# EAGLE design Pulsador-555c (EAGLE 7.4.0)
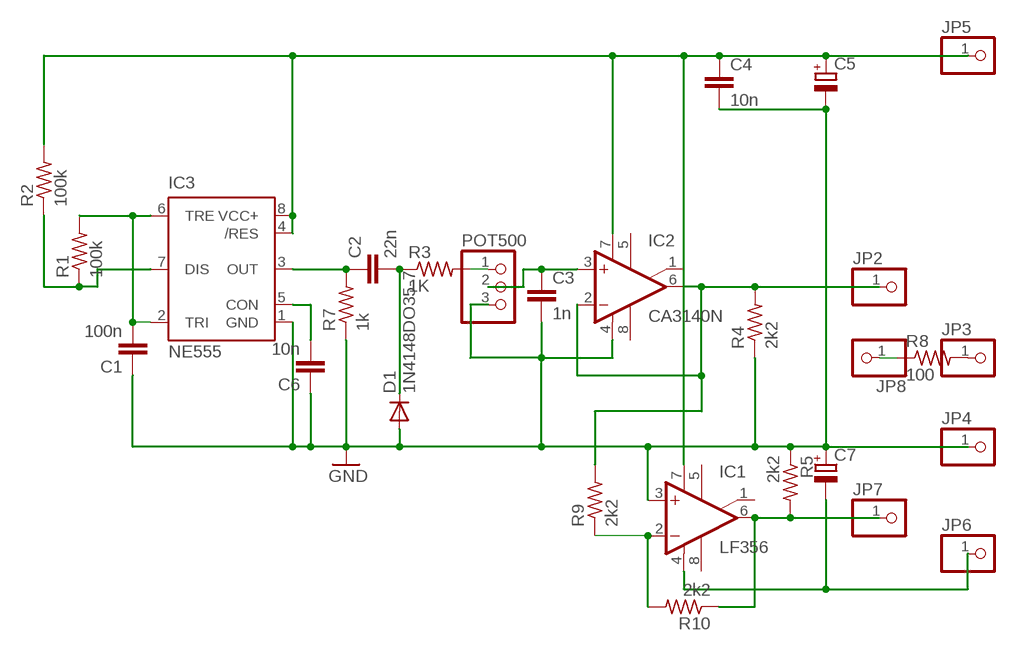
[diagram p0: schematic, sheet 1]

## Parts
C1  100n  C-EU050-024X044  [C050-024X044]
C2  22n  C-EU050-024X044  [C050-024X044]
C3  1n  C-EU050-024X044  [C050-024X044]
C4  10n  C-EU025-025X050  [C025-025X050]
C5  CPOL-EUE2.5-6  [E2,5-6]
C6  10n  C-EU050-024X044  [C050-024X044]
C7  CPOL-EUE2.5-6  [E2,5-6]
D1  1N4148DO35-7  [DO35-7]
IC1  LF356  CA3140N  [DIL08]
IC2  CA3140N  [DIL08]
IC3  NE555  [DIL-08]
JP2  PINHD-1X1  [1X01]
JP3  PINHD-1X1  [1X01]
JP4  PINHD-1X1  [1X01]
JP5  PINHD-1X1  [1X01]
JP6  PINHD-1X1  [1X01]
JP7  PINHD-1X1  [1X01]
JP8  PINHD-1X1  [1X01]
POT500  PINHD-1X3  [1X03]
R1  100k  R-US_0204/7  [0204/7]
R2  100k  R-US_0204/7  [0204/7]
R3  1K  R-US_0204/7  [0204/7]
R4  2k2  R-US_0204/7  [0204/7]
R5  2k2  R-US_0204/7  [0204/7]
R7  1k  R-US_0204/7  [0204/7]
R8  100  R-US_0204/7  [0204/7]
R9  2k2  R-US_0204/7  [0204/7]
R10  2k2  R-US_0204/7  [0204/7]

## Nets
GND: C1.1 C3.2 C4.2 C5.- C6.1 C7.+ D1.A IC1.3(+IN) IC2.4(V-) IC3.1(GND) JP4.1 POT500.3 R4.1 R5.1 R7.1
N$1: IC1.2(-IN) R9.1 R10.2
N$2: C6.2 IC3.5(CON)
N$3: C2.1 IC3.3(OUT) R7.2
N$4: C2.2 D1.C R3.1
N$5: C7.- IC1.4(V-) JP6.1
N$6: POT500.1 R3.2
N$7: IC2.2(-IN) IC2.6(OUT) JP2.1 R4.2 R9.2
N$9: IC3.7(DIS) R1.1 R2.1
N$10: C4.1 C5.+ IC1.7(V+) IC2.7(V+) IC3.4(/RES) IC3.8(VCC+) JP5.1 R2.2
N$11: C1.2 IC3.2(TRI) IC3.6(TRE) R1.2
N$12: JP3.1 R8.2
N$13: IC1.6(OUT) JP7.1 R5.2 R10.1
N$14: JP8.1 R8.1
N$16: C3.1 IC2.3(+IN) POT500.2
Unconnected: IC1.1(ON/CMP) IC1.5(ON) IC1.8(CMP) IC2.1(ON/CMP) IC2.5(ON) IC2.8(CMP)

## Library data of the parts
C1-C4 C6 = rcl:C-EU: CAPACITOR, European symbol
C5 C7 = rcl:CPOL-EU: POLARIZED CAPACITOR, European symbol
D1 = diode:1N4148: DIODE
IC1 IC2 = linear:CA3140: OP AMP
IC3 = st-microelectronics:NE555: General purpose bipolar Timer; MF: Arrow Electronics; MPN: NE555N; OC_FARNELL: 1467742; OC_NEWARK: 89K1486
JP2-JP8 = pinhead:PINHD-1X1: PIN HEADER
POT500 = pinhead:PINHD-1X3: PIN HEADER
R1-R5 R7-R10 = rcl:R-US_: RESISTOR, American symbol

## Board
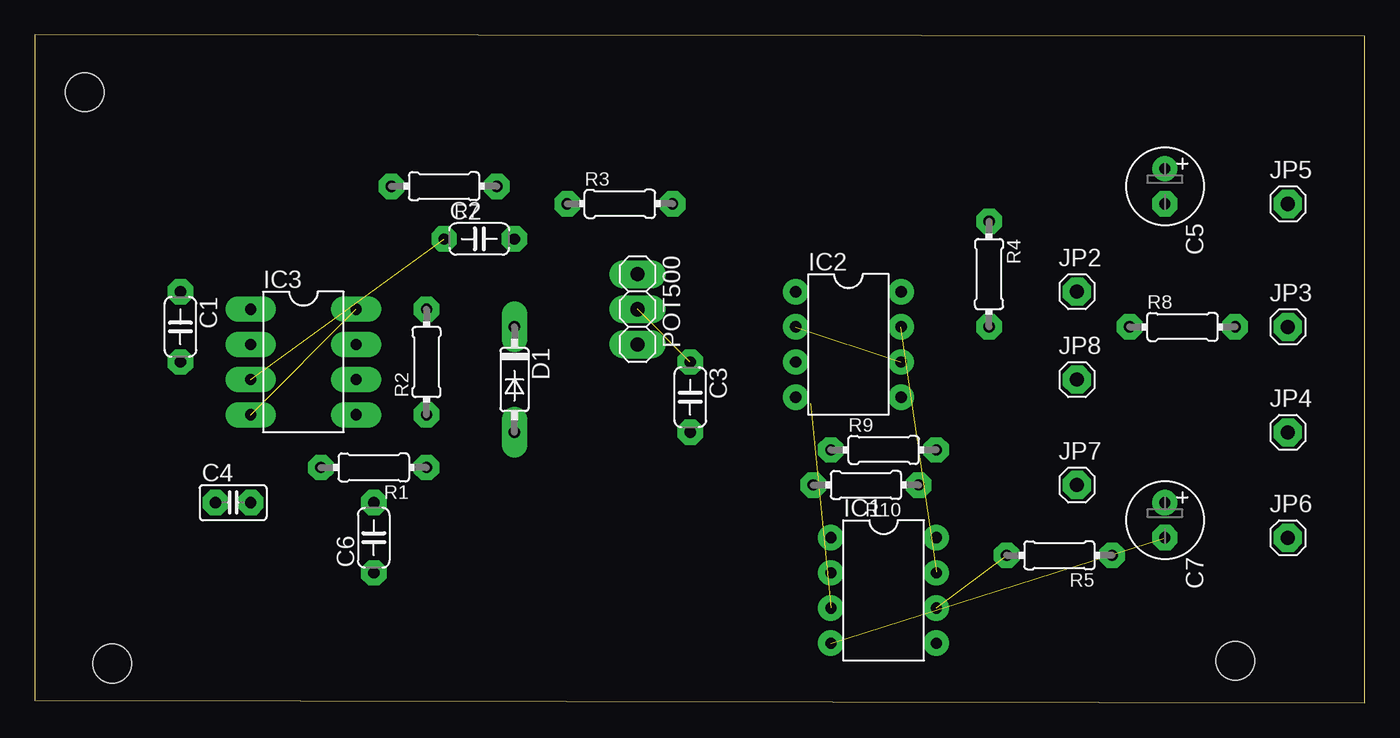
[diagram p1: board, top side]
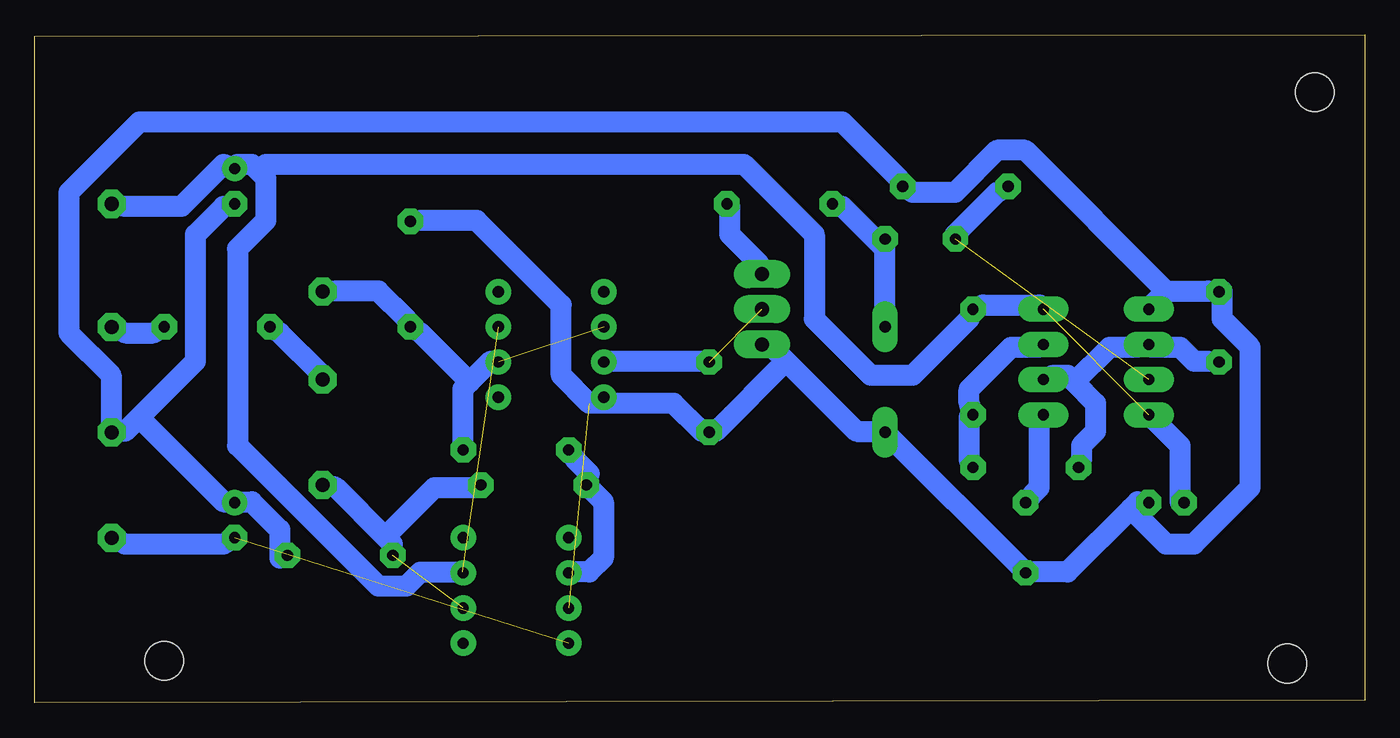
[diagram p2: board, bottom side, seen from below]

Size 96.1 x 48.3 mm. Coordinates in mm from the lower left corner, seen from the top.
Outline: 0,0.2 96.1,0 96.1,48.2 0,48.3 0,0.2
Copper layers (1*16): Top 0.035mm / dielectric 1.5mm / Bottom 0.035mm
Design rules "default *": minimum track width 60mil, minimum drill 24mil, track to track 20mil, track to pad 20mil, pad to pad 8mil, via to via 8mil, smd to smd 8mil, copper to edge 40mil, drill to drill 8mil, minimum pad ring 20mil, minimum via ring 8mil, stop-mask expansion 4mil, vias tented up to drill 0mil, thermal gap 10mil
Holes 2.8 mm at 3.61,44.15 86.73,3.05 5.61,2.85

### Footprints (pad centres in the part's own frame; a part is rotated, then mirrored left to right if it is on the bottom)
C050-024X044 = drill 0.813 octagon: 1 -2.54,0; 2 2.54,0
C025-025X050 = drill 0.813 octagon: 1 -1.27,0; 2 1.27,0
E2,5-6 = drill 0.813 pad 1.6: + -1.27,0 | drill 0.813 pad 1.6 octagon: - 1.27,0
DO35-7 = drill 0.813 long: A 3.81,0; C -3.81,0
DIL08 = drill 0.813 pad 1.27: 1 -3.81,-3.81; 2 -1.27,-3.81; 3 1.27,-3.81; 4 3.81,-3.81; 5 3.81,3.81; 6 1.27,3.81; 7 -1.27,3.81; 8 -3.81,3.81
DIL-08 = drill 0.813 long: 1 -3.81,-3.81; 2 -1.27,-3.81; 3 1.27,-3.81; 4 3.81,-3.81; 5 3.81,3.81; 6 1.27,3.81; 7 -1.27,3.81; 8 -3.81,3.81
1X01 = drill 1.016 octagon: 1 0,0
1X03 = drill 1.016 long: 1 -2.54,0; 2 0,0; 3 2.54,0
0204/7 = drill 0.813 octagon: 1 -3.81,0; 2 3.81,0

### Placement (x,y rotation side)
C1  10.53,27.18 270 top
C2  32.12,33.53 0 top
C3  47.36,22.1 270 top
C4  14.34,14.48 0 top
C5  81.65,37.34 270 top
C6  24.5,11.94 90 top
C7  81.65,13.21 270 top
D1  34.66,23.37 270 top
IC1  61.33,8.13 270 top
IC2  58.79,25.91 270 top
IC3  19.42,24.64 270 top
JP2  75.3,29.72 0 top
JP3  90.54,27.18 0 top
JP4  90.54,19.56 0 top
JP5  90.54,36.07 0 top
JP6  90.54,11.94 0 top
JP7  75.3,15.75 0 top
JP8  75.3,23.37 0 top
POT500  43.55,28.45 270 top
R1  24.5,17.02 180 top
R2  28.31,24.64 90 top
R3  42.28,36.07 0 top
R4  68.95,30.99 270 top
R5  74.03,10.67 180 top
R7  29.58,37.34 180 top
R8  82.92,27.18 0 top
R9  61.33,18.29 0 top
R10  60.06,15.75 180 top

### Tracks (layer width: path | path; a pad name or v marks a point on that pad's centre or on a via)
GND  (1 unrouted)
  Bottom 1.524: R5.1 78.38,10.48 78.38,12.51 80.42,14.54 81.43,14.54 C7.+ 82.45,14.54 88.54,20.64 | 88.54,20.64 89.56,19.62 JP4.1 90.58,19.62 90.58,23.69 93.62,26.74 93.62,36.9 88.54,41.98 37.74,41.98 33.68,37.91 R7.1 32.66,36.9 29.62,36.9 26.57,39.94 24.54,39.94 14.38,29.78 | 88.54,20.64 84.48,24.7 84.48,33.85 82.45,35.88 C5.- | 14.38,29.78 11.33,29.78 C1.1 10.31,29.78 10.31,27.75 8.28,25.72 8.28,15.56 12.34,11.5 14.38,11.5 16.92,14.04 | 14.38,29.78 15.39,28.77 IC3.1 | 24.54,9.46 21.49,9.46 16.92,14.04 | 16.92,14.04 16.41,14.54 C4.2 | 34.7,19.62 36.73,19.62 41.81,24.7 | 41.81,24.7 42.82,25.72 POT500.3 | 41.81,24.7 46.89,19.62 C3.2 47.9,19.62 49.94,21.66 55.02,21.66 | 55.02,21.66 56.03,21.66 58.06,23.69 58.06,28.77 64.16,34.86 68.22,34.86 R4.1 | 55.02,21.66 IC2.4 | 34.7,19.62 24.54,9.46 | 24.54,9.46 C6.1 | 34.7,19.62 D1.A
N$1
  Bottom 1.524: R9.1 57.05,17.59 56.03,16.58 R10.2 56.03,15.56 55.02,14.54 55.02,10.48 56.03,9.46 57.05,9.46 IC1.2
N$2
  Bottom 1.524: IC3.5 23.52,20.64 23.52,15.56 24.54,14.54 C6.2
N$3  (1 unrouted)
  Bottom 1.524: R7.2 26.57,36.9 29.62,33.85 C2.1
N$4
  Bottom 1.524: 34.7,32.83 34.7,27.75 D1.C | 34.7,32.83 37.74,35.88 R3.1 | 34.7,32.83 C2.2
N$5  (1 unrouted)
  Bottom 1.524: C7.- 82.45,11.5 89.56,11.5 JP6.1
N$6
  Bottom 1.524: R3.2 45.87,35.88 45.87,33.85 43.84,31.82 POT500.1
N$7  (1 unrouted)
  Bottom 1.524: 64.67,23.18 63.14,24.7 IC2.6 | 64.67,23.18 65.18,22.67 65.18,18.61 R9.2 | 64.67,23.18 68.22,26.74 R4.2 69.24,27.75 71.27,29.78 74.32,29.78 JP2.1
N$9
  Bottom 1.524: R1.1 28.6,17.59 28.6,20.64 R2.1 28.6,21.66 28.6,22.67 25.55,25.72 23.52,25.72 IC3.7
N$10  (2 unrouted)
  Bottom 1.524: C4.1 13.36,14.54 13.36,18.61 15.39,20.64 IC3.4 | IC3.8 23.52,28.77 27.58,28.77 R2.2 28.6,27.75 32.66,23.69 35.71,23.69 39.78,27.75 39.78,33.85 44.86,38.93 79.4,38.93 79.91,38.42 | 79.91,38.42 80.42,38.93 81.43,38.93 C5.+ 82.45,38.93 85.5,35.88 89.56,35.88 JP5.1 | 79.91,38.42 79.4,37.91 79.4,34.86 81.43,32.83 81.43,18.61 71.27,8.45 69.24,8.45 68.22,9.46 65.18,9.46 IC1.7
N$11
  Bottom 1.524: C1.2 11.33,24.7 12.34,24.7 13.36,25.72 15.39,25.72 IC3.2 16.41,25.72 18.44,25.72 20.98,23.18 | 20.98,23.18 21.49,23.69 22.5,23.69 IC3.6 | 20.98,23.18 19.46,21.66 19.46,19.62 20.47,18.61 20.47,17.59 R1.2
N$12
  Bottom 1.524: R8.2 87.53,26.74 89.56,26.74 JP3.1
N$13  (1 unrouted)
  Bottom 1.524: 70.76,12 74.32,15.56 JP7.1 | 70.76,12 70.26,11.5 R5.2 | 70.76,12 67.21,15.56 64.16,15.56 R10.1
N$14
  Bottom 1.524: R8.1 78.38,26.74 75.34,23.69 JP8.1
N$16  (1 unrouted)
  Bottom 1.524: C3.1 47.9,24.7 55.02,24.7 IC2.3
